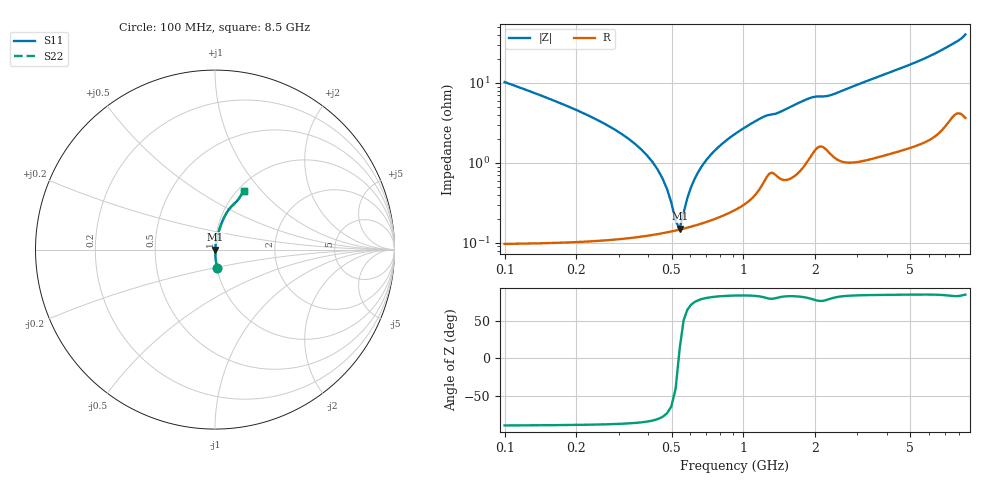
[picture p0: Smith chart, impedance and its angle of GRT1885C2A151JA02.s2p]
!Murata Part Number: GRT1885C2A151JA02
!These Parameters are Measured in Series Mode Connection
!Data Generated on Jun 19, 2026
!  o--ll--o
!Port1  Port2
!  o------o
!Operation Temp=25[degC], DC Bias Voltage=0[V]
!Freq. Start=100[MHz] Stop=9[GHz] 401[Steps]
# Hz S RI R 50
!Freq.(Hz) S11(Real) S11(Imag) S21(Real) S21(Imag) S12(Real) S12(Imag) S22(Real) S22(Imag)
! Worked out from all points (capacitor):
!   401 points, 100 MHz to 8.5 GHz, reference 50 ohm
!   read as one part in series: C = 150 pF near 142 MHz
!   lowest |Z| = 150 mohm at 541 MHz (marker M1)
!   series resonance near 536.4 MHz, so ESL is about 590 pH
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1e8  0.0113 -0.1012  0.9887 0.1012  0.9887 0.1012  0.0113 -0.1012
3.73e8  0.00141 -0.0147  0.9986 0.0147  0.9986 0.0147  0.00141 -0.0147
4.36e8  0.00135 -0.00824  0.9987 0.00824  0.9987 0.00824  0.00135 -0.00824
4.57e8  0.00135 -0.00635  0.9986 0.00635  0.9986 0.00635  0.00135 -0.00635
4.99e8  0.00139 -0.00285  0.9986 0.00285  0.9986 0.00285  0.00139 -0.00285
5.2e8  0.00142 -0.00122  0.9986 0.00122  0.9986 0.00122  0.00142 -0.00122
5.41e8  0.00146 0.000347  0.9985 -0.000347  0.9985 -0.000347  0.00146 0.000347
5.62e8  0.00151 0.00185  0.9985 -0.00185  0.9985 -0.00185  0.00151 0.00185
6.25e8  0.00167 0.00609  0.9983 -0.00609  0.9983 -0.00609  0.00167 0.00609
6.67e8  0.00181 0.00871  0.9982 -0.00871  0.9982 -0.00871  0.00181 0.00871
7.3e8  0.00206 0.0124  0.9979 -0.0124  0.9979 -0.0124  0.00206 0.0124
8.14e8  0.00245 0.0171  0.9976 -0.0171  0.9976 -0.0171  0.00245 0.0171
9.61e8  0.00335 0.0247  0.9966 -0.0247  0.9966 -0.0247  0.00335 0.0247
1.15e9  0.00552 0.034  0.9945 -0.034  0.9945 -0.034  0.00552 0.034
1.507e9  0.0082 0.046  0.9918 -0.046  0.9918 -0.046  0.0082 0.046
1.906e9  0.0156 0.062  0.9844 -0.062  0.9844 -0.062  0.0156 0.062
2.284e9  0.0177 0.0659  0.9823 -0.0659  0.9823 -0.0659  0.0177 0.0659
2.914e9  0.018 0.0887  0.982 -0.0887  0.982 -0.0887  0.018 0.0887
4.3e9  0.0322 0.1354  0.9678 -0.1354  0.9678 -0.1354  0.0322 0.1354
5.707e9  0.054 0.1858  0.946 -0.1858  0.946 -0.1858  0.054 0.1858
7.114e9  0.0954 0.2442  0.9046 -0.2442  0.9046 -0.2442  0.0954 0.2442
8.5e9  0.1608 0.3248  0.8392 -0.3248  0.8392 -0.3248  0.1608 0.3248
